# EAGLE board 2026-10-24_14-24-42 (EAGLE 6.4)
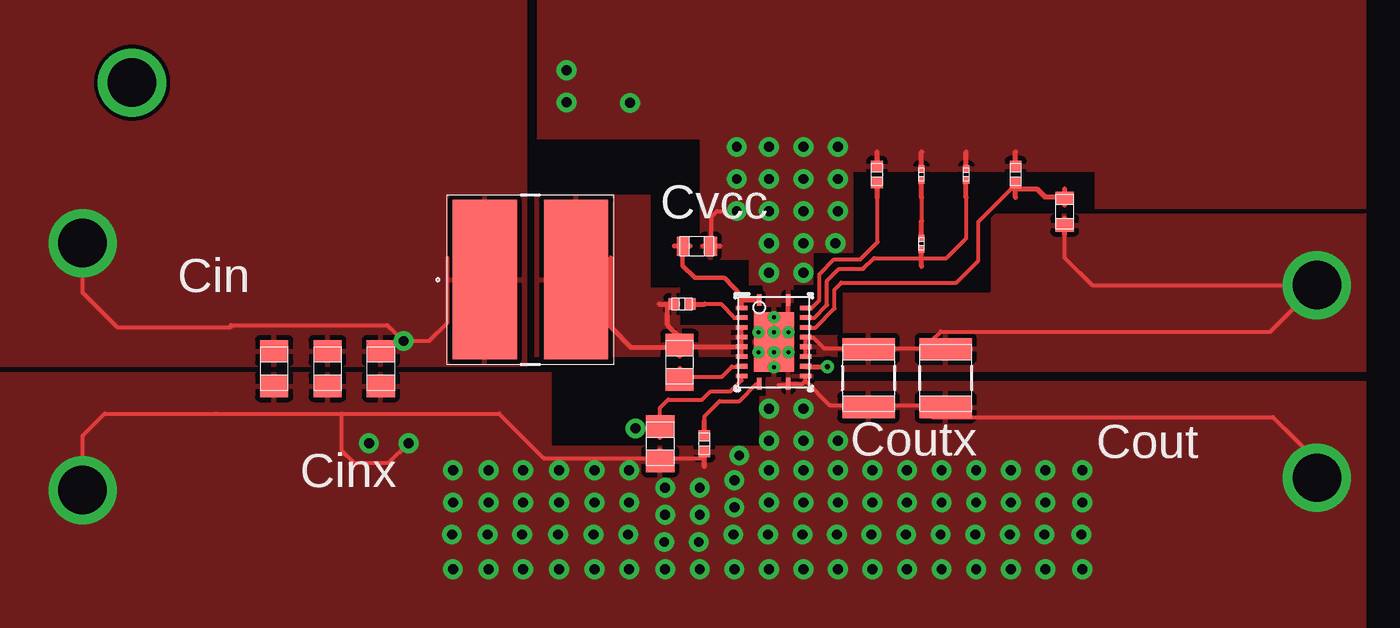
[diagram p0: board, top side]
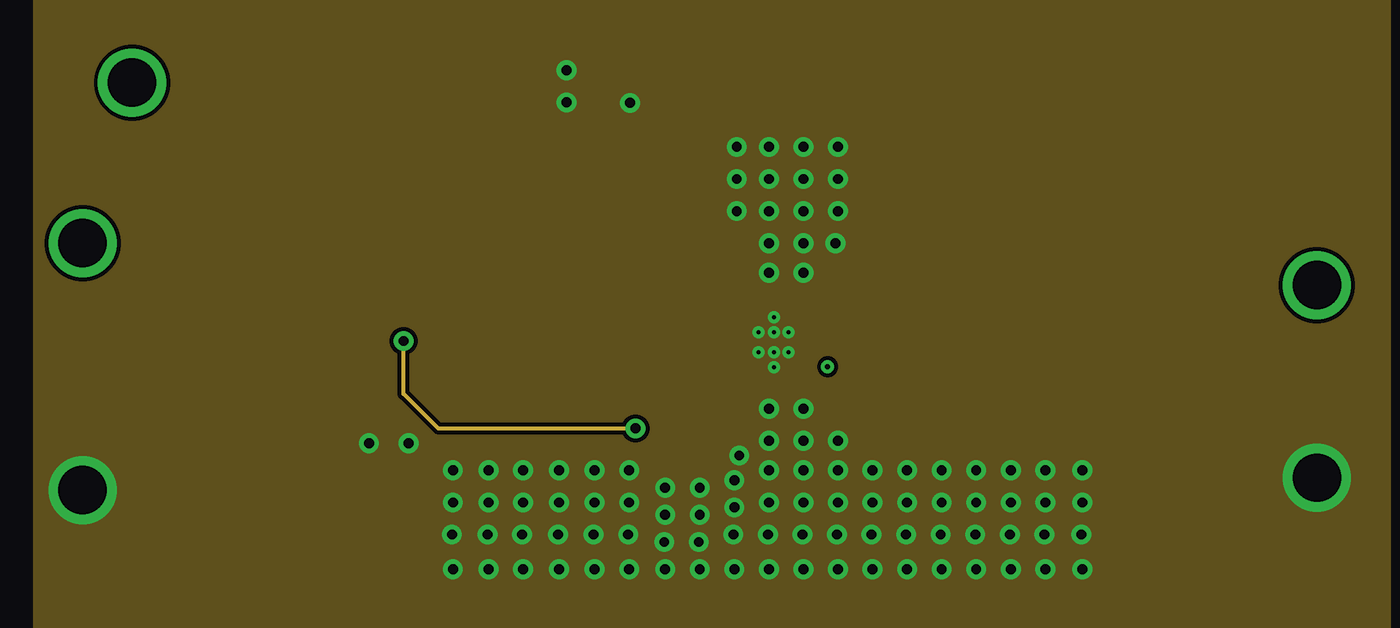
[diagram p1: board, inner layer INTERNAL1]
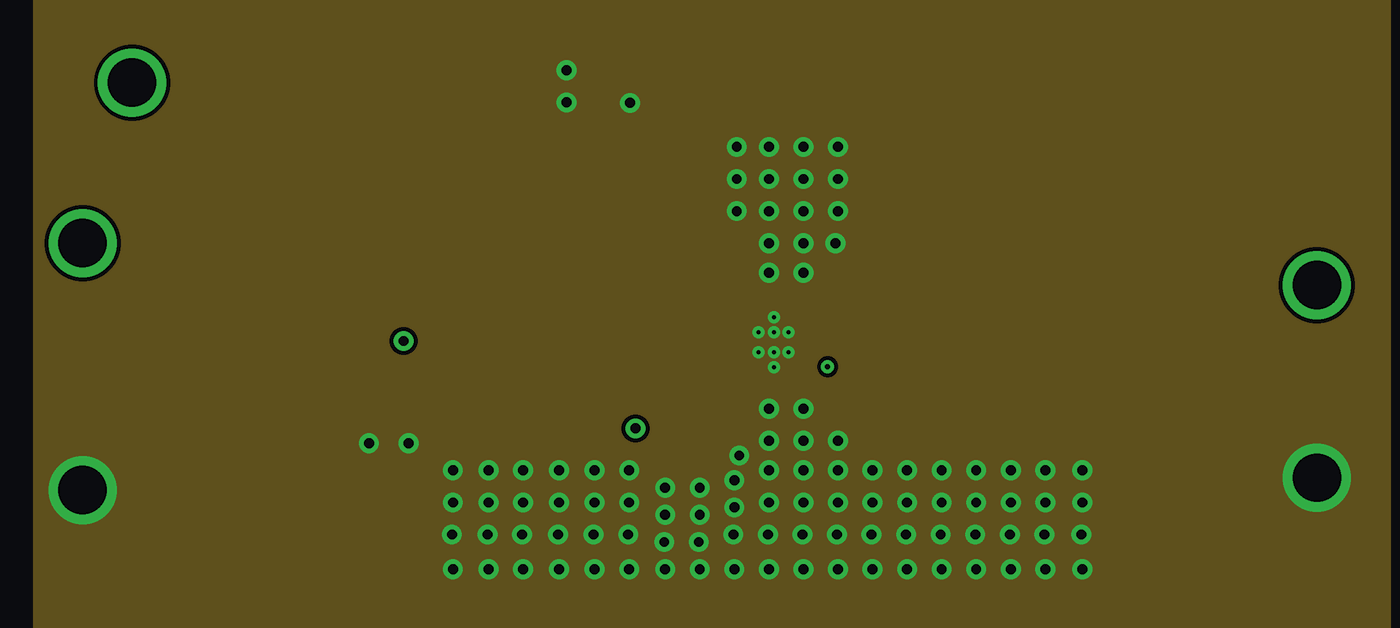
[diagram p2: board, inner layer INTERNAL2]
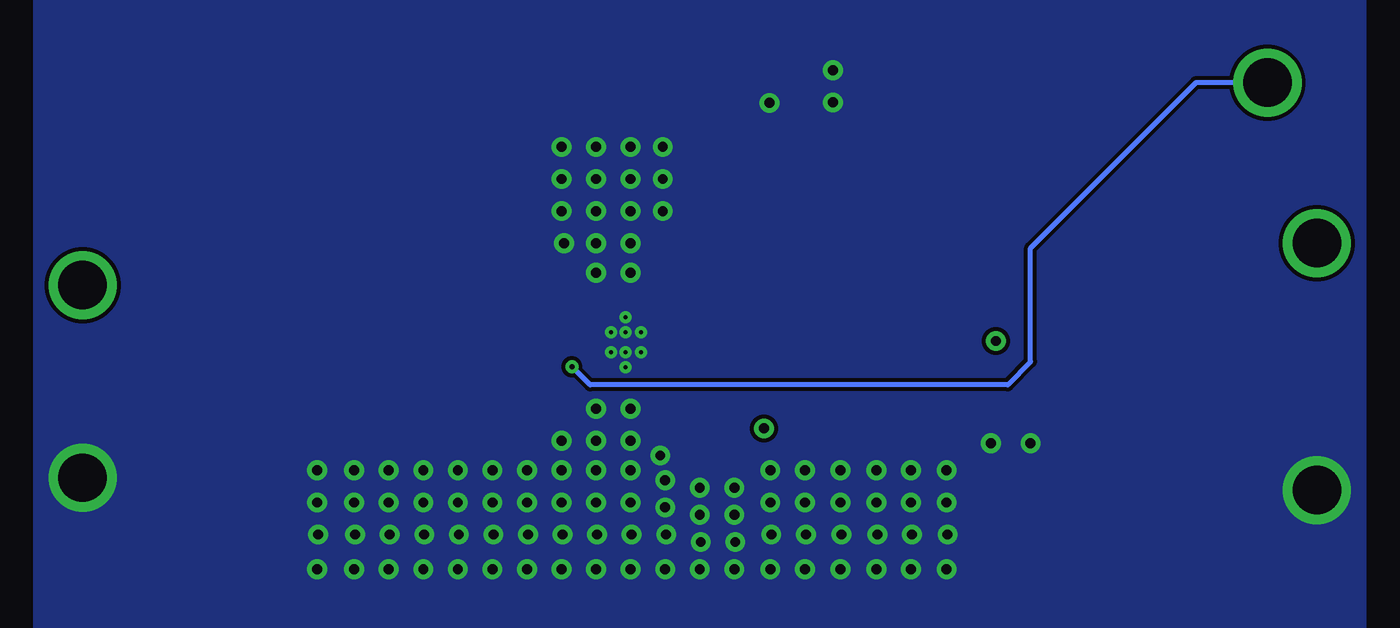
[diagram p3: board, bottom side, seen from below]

No outline drawn. Coordinates in mm, seen from the top.
Copper layers ((1*2)+(15*16)): TOP / INTERNAL1 / layer 15 / BOTTOM

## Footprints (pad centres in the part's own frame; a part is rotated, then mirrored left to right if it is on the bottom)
0805 = smd 1.118 x 1.448: 1 -0.902,0; 2 0.902,0
0201 = smd 0.356 x 0.33: 1 -0.292,0; 2 0.292,0
1210_280 = smd 1.118 x 2.692: 1 -1.499,0; 2 1.499,0
0402 = smd 0.559 x 0.61: 1 -0.419,0; 2 0.419,0
0603 = smd 0.66 x 0.965: 1 -0.699,0; 2 0.699,0
TP-1502 = drill 0.813 pad 1.651 round: 1 0,0
VLP8040 = smd 3.302 x 8.204: 1 -2.349,0; 2 2.349,0
RHL0020A = smd 0.24 x 0.6: 1 -0.75,2.15; 10 -0.75,-2.15; 11 0.75,-2.15; 20 0.75,2.15 | smd 0.6 x 0.24: 2 -1.65,1.75; 3 -1.65,1.25; 4 -1.65,0.75; 5 -1.65,0.25; 6 -1.65,-0.25; 7 -1.65,-0.75; 8 -1.65,-1.25; 9 -1.65,-1.75; 12 1.65,-1.75; 13 1.65,-1.25; 14 1.65,-0.75; 15 1.65,-0.25; 16 1.65,0.25; 17 1.65,0.75; 18 1.65,1.25; 19 1.65,1.75 | smd 2.05 x 3.05: 21 0,0

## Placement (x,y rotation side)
Cbst  [0805]  61.19,52.3 270 top
Ccomp  [0201]  73.63,61.95 90 top
Ccomp2  [0201]  75.95,61.95 90 top
Cin2  [0805]  60.2,48.11 270 top
Cin_1  [0805]  45.82,51.97 270 top
Cin_2  [0805]  43.08,51.97 270 top
Cin_3  [0805]  40.34,51.97 270 top
Cout_1  [1210_280]  70.92,51.49 270 top
Cout_2  [1210_280]  74.88,51.49 270 top
Css  [0402]  62.46,48.11 270 top
Cvcc_1  [0603]  62.08,58.27 0 top
Cvcc_2  [0603]  62.08,58.27 0 top
GND  [TP-1502]  30.45,45.69 0 top
GND1  [TP-1502]  93.95,46.33 0 top
L1  [VLP8040]  53.52,56.54 0 top
MODE  [TP-1502]  32.99,66.67 0 top
Rcomp  [0201]  73.63,58.39 90 top
Rfbb  [0402]  78.49,61.95 90 top
Rfbt  [0603]  81,60.05 90 top
Rlim  [0402]  71.35,61.95 90 top
Rt  [0402]  61.32,55.3 0 top
U1  [RHL0020A]  66.04,53.34 0 top
VIN  [TP-1502]  30.45,58.39 0 top
VOUT  [TP-1502]  93.95,56.24 0 top

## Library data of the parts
Cbst = ultra-librarian; RefDes: Cbst; Type: 08053C104KAT2A
Ccomp = ultra-librarian; RefDes: Ccomp; Type: GRM033R71C681KA01D
Ccomp2 = ultra-librarian; RefDes: Ccomp2; Type: CGA1A2C0G1E330J030BA
Cin2 = ultra-librarian; RefDes: Cin2; Type: 08053C104KAT2A
Cin_1-Cin_3 Cout_1 Cout_2 Cvcc_1 Cvcc_2 = ultra-librarian
Css = ultra-librarian; RefDes: Css; Type: GRM155R71C822KA01D
GND = ultra-librarian; RefDes: GND; Type: TP-1502
GND1 = ultra-librarian; RefDes: GND1; Type: TP-1502
L1 = ultra-librarian; RefDes: L1; Type: VLP8040T-1R0N
MODE = ultra-librarian; RefDes: MODE; Type: TP-1502
Rcomp = ultra-librarian; RefDes: Rcomp; Type: RC0201FR-0728K7L
Rfbb = ultra-librarian; RefDes: Rfbb; Type: CRCW040269K8FKED
Rfbt = ultra-librarian; RefDes: Rfbt; Type: RC0603FR-07220KL
Rlim = ultra-librarian; RefDes: Rlim; Type: CRCW040269K8FKED
Rt = ultra-librarian; RefDes: Rt; Type: CRCW0402267KFKED
U1 = ultra-librarian; RefDes: U1; Type: TPS61088QRHLRQ1
VIN = ultra-librarian; RefDes: VIN; Type: TP-1502
VOUT = ultra-librarian; RefDes: VOUT; Type: TP-1502

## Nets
0: Ccomp2.2 Ccomp.2 Cin2.2 Cin_1.2 Cin_2.2 Cin_3.2 Cout_1.2 Cout_2.2 Css.2 Cvcc_1.2 Cvcc_2.2 GND1.1 GND.1 Rfbb.2 Rlim.2 U1.11 U1.12 U1.20 U1.21
2: Cin2.1 Cin_1.1 Cin_2.1 Cin_3.1 L1.1 U1.9 VIN.1
3: Ccomp.1 Rcomp.2
4: Cvcc_1.1 Cvcc_2.1 U1.1 U1.2
5: Ccomp2.1 Rcomp.1 U1.18
9: Cout_1.1 Cout_2.1 Rfbt.1 U1.14 U1.15 U1.16 VOUT.1
11: Rfbb.1 Rfbt.2 U1.17
12: Cbst.1 L1.2 Rt.1 U1.4 U1.5 U1.6 U1.7
14: Rlim.1 U1.19
15: Rt.2 U1.3
17: MODE.1 U1.13
19: Css.1 U1.10
21: Cbst.2 U1.8

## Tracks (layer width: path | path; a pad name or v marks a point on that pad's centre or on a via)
0  (via drill 0.2 pad 0.48, 0.51 pad 1.02, 2.49 pad 3.48)
  TOP 0.203: v66.04,54.61 66.78,54.61 66.78,55.47 | 43.81,49.66 43.81,47.75 44.45,47.12 46.23,47.12 v47.24,48.13 | 43.81,49.66 37.34,49.66 31.62,49.66 30.48,48.51 v30.48,45.72 | v93.98,46.35 93.98,47.24 91.72,49.48 74.19,49.48 73.58,50.09 71.14,50.09 | 62.48,47.37 60.2,47.37 54.2,47.37 51.92,49.66 43.81,49.66 | v64.14,60.07 63.12,60.07 62.84,59.79 62.84,58.29 | 67.67,51.33 67.51,51.18 66.78,51.18 66.75,51.13 66.29,51.13 | 70.94,50.29 71.14,50.09 | 67.67,51.33 68.91,50.09 71.14,50.09 | 67.67,51.33 | 67.67,51.33 67.67,51.59
  TOP 0.254: 60.19,46.94 60.19,47.78 | 78.47,62.28 78.47,63.12 | 62.47,46.94 62.47,47.78 | 71.36,62.28 71.36,63.12 | 75.93,62.28 75.93,63.12 | 73.65,62.28 73.65,63.12 | 62.41,58.28 63.25,58.28
  other vias: 49.53,41.66 67.56,41.66 65.79,41.66 78.23,41.66 76.45,41.66 80.01,41.66 72.9,41.66 71.12,41.66 74.68,41.66 69.34,41.66 64.01,41.66 81.92,41.66 60.45,41.66 62.23,41.66 56.82,41.66 58.6,41.66 53.14,41.66 51.36,41.66 54.99,41.66 65.79,49.91 67.56,49.91 67.56,48.26 65.79,48.26 67.56,46.74 65.79,46.74 67.56,45.09 65.79,45.09 69.34,48.26 69.34,46.74 74.68,46.74 71.12,46.74 72.9,46.74 80.01,46.74 76.45,46.74 78.23,46.74 78.23,45.09 80.01,45.09 72.9,45.09 71.12,45.09 69.34,45.09 64.01,44.83 64.01,46.23 64.26,47.5 81.92,45.09 81.92,46.74 45.21,48.13 65.79,56.9 67.56,56.9 65.79,58.42 67.56,58.42 67.56,60.07 65.79,60.07 69.34,60.07 69.34,61.72 64.14,61.72 65.79,61.72 67.56,61.72 67.56,63.37 65.79,63.37 64.14,63.37 69.34,63.37 60.45,44.45 62.23,44.45 56.82,45.09 58.6,45.09 58.65,65.63 55.37,67.31 55.37,65.66 69.22,58.42 58.6,46.74 56.82,46.74 62.23,45.85 60.45,45.85 54.99,46.74 51.36,46.74 53.14,46.74 53.14,45.09 51.36,45.09 54.99,45.09 54.94,43.43 51.31,43.43 53.09,43.43 58.55,43.43 56.77,43.43 62.18,43.05 60.4,43.05 81.86,43.43 63.96,43.43 69.29,43.43 74.63,43.43 71.07,43.43 72.85,43.43 79.96,43.43 76.4,43.43 78.18,43.43 65.74,43.43 67.51,43.43 49.48,43.43 49.53,45.09 49.53,46.74 66.8,53.85 66.04,53.85 66.04,52.04 65.25,53.85 74.68,45.09 76.45,45.09 65.25,52.81 66.04,52.81 66.8,52.81
  pour TOP (rank 4): 65.05,51.74 65.61,51.74 65.61,50.93 65.71,50.83 65.81,50.83 65.91,50.93 65.91,51.36 66.14,51.36 66.14,50.93 66.24,50.83 66.34,50.83 66.45,50.93 66.45,51.74 67.01,51.74 67.11,51.84 67.11,54.81 67.01,54.91 66.45,54.91 66.45,55.73 66.34,55.83 66.24,55.83 66.14,55.73 66.14,55.3 65.91,55.3 65.91,55.73 65.81,55.83 65.71,55.83 65.61,55.73 65.61,54.91 65.05,54.91 64.95,54.81 64.95,51.84
  pour TOP: 64.77,56.26 65.48,56.26 65.48,55.09 64.97,55.09 64.97,51.79 65.63,51.79 65.63,50.55 65.3,50.55 65.3,48.01 54.61,48.01 54.61,51.79 26.04,51.79 26.04,30.48 96.52,30.48 96.52,51.31 68.07,51.31 68.07,51.69 67.06,51.69 67.06,56.29 68.07,56.29 68.07,57.94 70.1,57.94 70.1,62.1 82.55,62.1 82.55,60.2 96.52,60.2 96.52,76.2 53.85,76.2 53.85,63.75 62.23,63.75 62.23,57.56 64.77,57.56
  pour BOTTOM (rank 5): 27.94,76.2 96.52,76.2 96.52,30.48 27.94,30.48
  pour INTERNAL2 (rank 6): 27.94,77.47 97.79,77.47 97.79,29.21 27.94,29.21
  pour INTERNAL1: 27.94,77.47 97.79,77.47 97.79,29.21 27.94,29.21
2  (via drill 0.51 pad 1.02, 2.49 pad 3.48)
  TOP 0.203: 49.25,57.66 49.25,54.33 48.31,53.39 v46.99,53.39 | v30.48,58.42 30.48,55.88 32.26,54.1 38.1,54.1 38.1,54.2 46.15,54.2 v46.99,53.39 | U1.9 64.39,51.36 63.8,50.8 62.79,50.8 62.36,50.37 60.6,50.37 60.2,49.96 60.2,48.87 58.93,48.87 v58.93,48.9 | v46.99,53.39 | v46.99,53.39
  TOP 0.254: 60.19,48.44 60.19,49.28
  INTERNAL1 0.203: v46.99,53.39 46.99,50.67 48.77,48.9 v58.93,48.9
  pour TOP (rank 3): 26.04,76.2 53.34,76.2 53.34,52.07 26.04,52.07
3
  TOP 0.203: 73.66,59.16 73.66,61.21 | 73.66,59.16
  TOP 0.254: 73.65,60.78 73.65,61.62 | 73.65,58.73 73.65,59.56
4
  TOP 0.229: 61.34,58.29 61.34,57.25 61.98,56.64 63.5,56.64 64.39,55.73 64.39,55.4 | 65.28,55.47 64.44,55.47 64.39,55.4 | 64.39,55.07 64.39,55.4
  TOP 0.254: 60.91,58.28 61.75,58.28
5
  TOP 0.203: 75.95,61.21 75.95,58.67 74.93,57.66 73.66,57.66 71.2,57.66 70.64,57.1 69.39,57.1 68.78,56.49 68.78,55.24 68.12,54.59 67.67,54.59
  TOP 0.254: 75.93,60.78 75.93,61.62 | 73.65,57.23 73.65,58.06
9  (via drill 2.49 pad 3.48)
  TOP 0.203: 81.03,59.31 81.03,57.66 82.42,56.26 v93.98,56.26 91.59,53.87 74.62,53.87 73.74,53.01 71.14,53.01 68.63,53.01 68.07,53.57 67.67,53.57 67.67,53.09 67.67,52.58
  TOP 0.254: 81.01,58.88 81.01,59.72
  pour TOP: 77.22,59.94 77.22,55.88 69.6,55.88 69.6,53.7 67.41,53.7 67.41,52.58 69.6,52.58 69.6,51.82 96.52,51.82 96.52,59.94
11
  TOP 0.203: 67.67,54.08 68.17,54.08 69.16,55.07 69.16,56.03 69.52,56.39 75.44,56.39 76.56,57.51 76.56,59.51 78.26,61.21 78.49,61.21
  TOP 0.254: 78.49,61.21 79.58,61.21 79.98,60.81 81.03,60.81 | 78.47,60.78 78.47,61.62 | 81.01,60.38 81.01,61.21
12
  TOP 0.203: 64.39,52.58 U1.6 64.39,53.57 64.39,54.08
  TOP 0.254: 57.66,57.66 57.66,54.1 58.67,53.06 61.21,53.06 | 60.58,55.3 60.58,54.2 61.21,53.59 61.21,53.06 | U1.6 61.21,53.09 61.21,53.06 | 60.15,55.28 60.98,55.28 | 61.2,52.63 61.2,53.47
  pour TOP (rank 2): 59.69,56.13 61.21,56.13 61.21,54.2 63.65,54.2 64.64,54.2 64.64,52.58 53.72,52.58 53.72,60.91 59.69,60.91
14
  TOP 0.203: 67.67,55.07 67.97,55.07 68.38,55.47 68.38,56.82 69.14,57.58 70.48,57.58 71.37,58.47 71.37,61.21
  TOP 0.254: 71.36,60.78 71.36,61.62
15
  TOP 0.203: 62.08,55.3 63.32,55.3 64.01,54.59 U1.3
  TOP 0.254: 61.65,55.28 62.48,55.28
17  (via drill 0.25 pad 0.51, 2.49 pad 3.48)
  TOP 0.254: 67.67,52.07 v68.81,52.07
  BOTTOM 0.254: 33.15,66.8 v33.02,66.67 36.7,66.67 45.21,58.17 45.21,52.32 46.38,51.13 67.87,51.13 v68.81,52.07
19
  TOP 0.203: 62.48,48.87 62.48,49.53 63.25,50.29 64.26,50.29 65.15,51.18 65.28,51.18
  TOP 0.254: 62.47,48.44 62.47,49.28
21
  TOP 0.203: 61.21,51.56 63.37,51.56 63.88,52.07 64.39,52.07
  TOP 0.254: 61.2,51.13 61.2,51.97

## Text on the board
ASSYNOTES: Cvcc | Cin | Coutx | Cout | Cinx | Note: | For PFM mode Connect mode TP to GND TP. | For PWM mode Connect mode TP to Vin TP.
